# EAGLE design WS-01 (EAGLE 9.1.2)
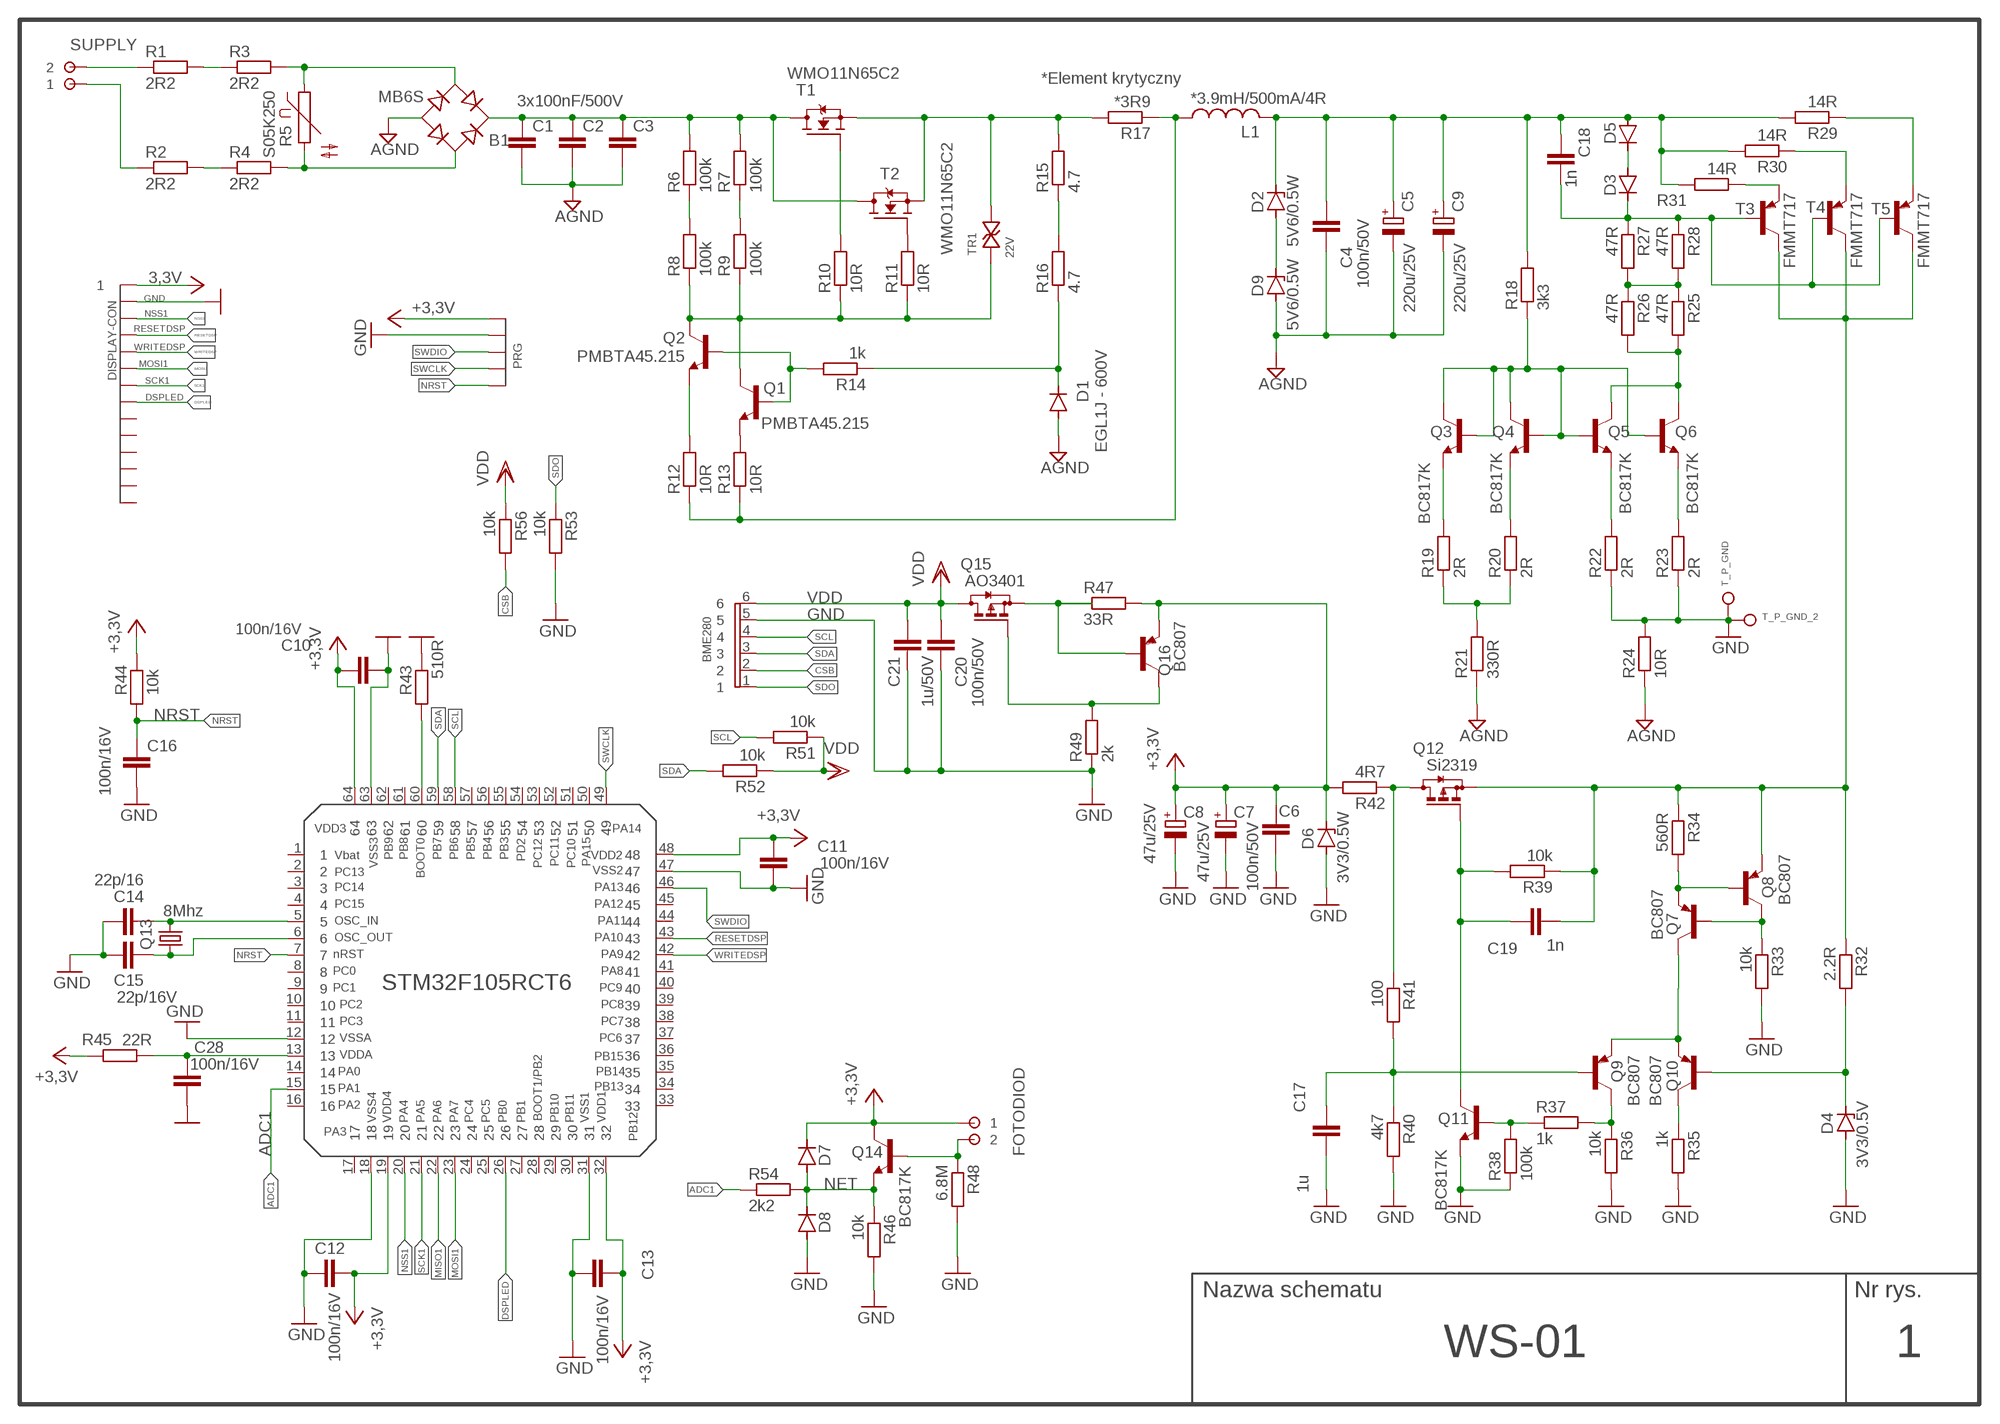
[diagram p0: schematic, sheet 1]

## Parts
B1  MB6S  [SOIC-4]
BME280  GOLDPIN6  [GOLDPIN6]
C1  3x100nF/500V  C-EUC1812  [C1812]
C2  C-EUC1812  [C1812]
C3  C-EUC1812  [C1812]
C4  100n/50V  C-EUC0805  [C0805]
C5  220u/25V  CPOL-EU175TMP-0810  [175TMP-0810]
C6  100n/50V  C-EUC0805  [C0805]
C7  47u/25V  CPOL-EU153CLV-0505  [153CLV-0505]
C8  47u/25V  CPOL-EU153CLV-0505  [153CLV-0505]
C9  220u/25V  CPOL-EU175TMP-0810  [175TMP-0810]
C10  100n/16V  C-EUC0805  [C0805]
C11  100n/16V  C-EUC0805  [C0805]
C12  100n/16V  C-EUC0805  [C0805]
C13  100n/16V  C-EUC0805  [C0805]
C14  22p/16  C-EUC0805  [C0805]
C15  22p/16V  C-EUC0805  [C0805]
C16  100n/16V  C-EUC0805  [C0805]
C17  1u  C-EUC0805  [C0805]
C18  1n  C-EUC0805  [C0805]
C19  1n  C-EUC0805  [C0805]
C20  100n/50V  C-EUC0805  [C0805]
C21  1u/50V  C-EUC0805  [C0805]
C28  100n/16V  C-EUC0805  [C0805]
D1  EGL1J - 600V  DIODE-MINIMELF  [MINIMELF]
D2  5V6/0.5W  ZENER-DIODESOD80C  [SOD80C]
D3  DIODE-MINIMELF  [MINIMELF]
D4  3V3/0.5V  ZENER-DIODESOD80C  [SOD80C]
D5  DIODE-MINIMELF  [MINIMELF]
D6  3V3/0.5W  ZENER-DIODESOD80C  [SOD80C]
D7  DIODE-MINIMELF  [MINIMELF]
D8  DIODE-MINIMELF  [MINIMELF]
D9  5V6/0.5W  ZENER-DIODESOD80C  [SOD80C]
DISPLAY-CON  GOLDPIN14  [GOLDPIN14]
FOTODIOD  ARK254  [ARK254]
L1  *3.9mH/500mA/4R  L-US6000-XXX-RC  [6000-XXXX-RC]
PRG  GOLDPIN5  [GOLDPIN5]
Q1  PMBTA45.215  BC847ASMD  [SOT23]
Q2  PMBTA45.215  BC847ASMD  [SOT23]
Q3  BC817K  BC817-16LT1SMD  [SOT23-BEC]
Q4  BC817K  BC817-16LT1SMD  [SOT23-BEC]
Q5  BC817K  BC817-16LT1SMD  [SOT23-BEC]
Q6  BC817K  BC817-16LT1SMD  [SOT23-BEC]
Q7  BC807  BC807-25SMD  [SOT23-BEC]
Q8  BC807  BC807-25SMD  [SOT23-BEC]
Q9  BC807  BC807-25SMD  [SOT23-BEC]
Q10  BC807  BC807-25SMD  [SOT23-BEC]
Q11  BC817K  BC817-16LT1SMD  [SOT23-BEC]
Q12  Si2319  BSS84  [SOT23]
Q13  8Mhz  CRYSTALHC49S  [HC49/S]
Q14  BC817K  BC817-16LT1SMD  [SOT23-BEC]
Q15  AO3401  BSS84  [SOT23]
Q16  BC807  BC807-25SMD  [SOT23-BEC]
R1  2R2  R-EU_R0805  [R0805]
R2  2R2  R-EU_R0805  [R0805]
R3  2R2  R-EU_R0805  [R0805]
R4  2R2  R-EU_R0805  [R0805]
R5  S05K250  [S05K250]
R6  100k  R-EU_R1206  [R1206]
R7  100k  R-EU_R1206  [R1206]
R8  100k  R-EU_R1206  [R1206]
R9  100k  R-EU_R1206  [R1206]
R10  10R  R-EU_R0805  [R0805]
R11  10R  R-EU_R0805  [R0805]
R12  10R  R-EU_R0805  [R0805]
R13  10R  R-EU_R0805  [R0805]
R14  1k  R-EU_R1206  [R1206]
R15  4.7  R-EU_R0805  [R0805]
R16  4.7  R-EU_R0805  [R0805]
R17  *3R9  R-EU_R1206  [R1206]
R18  3k3  R-EU_R0805  [R0805]
R19  2R  R-EU_R0805  [R0805]
R20  2R  R-EU_R0805  [R0805]
R21  330R  R-EU_R0805  [R0805]
R22  2R  R-EU_R0805  [R0805]
R23  2R  R-EU_R0805  [R0805]
R24  10R  R-EU_R1206  [R1206]
R25  47R  R-EU_R1206  [R1206]
R26  47R  R-EU_R1206  [R1206]
R27  47R  R-EU_R1206  [R1206]
R28  47R  R-EU_R1206  [R1206]
R29  14R  R-EU_R0805  [R0805]
R30  14R  R-EU_R0805  [R0805]
R31  14R  R-EU_R0805  [R0805]
R32  2.2R  R-EU_R0805  [R0805]
R33  10k  R-EU_R0805  [R0805]
R34  560R  R-EU_R0805  [R0805]
R35  1k  R-EU_R0805  [R0805]
R36  10k  R-EU_R0805  [R0805]
R37  1k  R-EU_R0805  [R0805]
R38  100k  R-EU_R0805  [R0805]
R39  10k  R-EU_R0805  [R0805]
R40  4k7  R-EU_R0805  [R0805]
R41  100  R-EU_R0805  [R0805]
R42  4R7  R-EU_R1206  [R1206]
R43  510R  R-EU_R0805  [R0805]
R44  10k  R-EU_R0805  [R0805]
R45  22R  R-EU_R0805  [R0805]
R46  10k  R-EU_R0805  [R0805]
R47  33R  R-EU_R0805  [R0805]
R48  6.8M  R-EU_R0805  [R0805]
R49  2k  R-EU_R0805  [R0805]
R51  10k  R-EU_R0805  [R0805]
R52  10k  R-EU_R0805  [R0805]
R53  10k  R-EU_R0805  [R0805]
R54  2k2  R-EU_R0805  [R0805]
R56  10k  R-EU_R0805  [R0805]
SUPPLY  ARK254  [ARK254]
T1  WMO11N65C2  MOS_TO252  [MOS_TO252]
T2  WMO11N65C2  MOS_TO252  [MOS_TO252]
T3  FMMT717  BC807-16-PNP-SOT23-BEC  [SOT23-BEC]
T4  FMMT717  BC807-16-PNP-SOT23-BEC  [SOT23-BEC]
T5  FMMT717  BC807-16-PNP-SOT23-BEC  [SOT23-BEC]
T_P_GND  PAD3  [PAD3]
T_P_GND_2  PAD3  [PAD3]
TR1  22V  SMAJ30CA-TR__DO214AC+MINIMELF  [DO214AC+MINIMELF_BIDIR]
U$2  STM32F105RCT6  [STM32F105RCT6]

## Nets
ADC1: R54.1 U$2.15
AGND: B1.- C1.2 C2.2 C3.2 C4.2 C5.- C9.- D1.A D9.A R21.1 R24.1
CSB: BME280.2 R56.2
DSPLED: DISPLAY-CON.8 U$2.26
GND: BME280.5 C6.2 C7.- C8.- C10.1 C11.1 C12.1 C13.2 C14.1 C15.1 C16.2 C17.2 C20.2 C21.2 C28.1 D4.A D6.A D8.A DISPLAY-CON.2 PRG.2 Q11.E R22.1 R23.1 R24.2 R33.2 R35.2 R36.2 R38.1 R40.2 R43.2 R46.2 R48.2 R49.1 R53.2 T_P_GND.P T_P_GND_2.P U$2.12 U$2.18 U$2.31 U$2.47 U$2.63
MISO1: U$2.22
MOSI1: DISPLAY-CON.6 U$2.23
N$1: R1.1 SUPPLY.2
N$2: R2.1 SUPPLY.1
N$3: R1.2 R3.1
N$4: R2.2 R4.1
N$5: B1.~2(AC2) R3.2 R5.1
N$6: B1.~1(AC1) R4.2 R5.2
N$7: B1.+ C1.1 C2.1 C3.1 R6.2 R7.2 T1.2(D) T2.2(D)
N$8: R6.1 R8.2
N$9: R7.1 R9.2
N$10: R15.2 R17.2 T1.3(S) T2.3(S) TR1.P$2
N$11: R11.2 T2.1(G)
N$12: Q1.3(C) Q2.3(C) R8.1 R9.1 R10.1 R11.1 TR1.P$1
N$13: Q1.1(B) Q2.1(B) R14.2
N$14: R10.2 T1.1(G)
N$15: Q1.2(E) R13.2
N$16: Q2.2(E) R12.2
N$17: L1.1 R12.1 R13.1 R17.1
N$18: R30.1 T4.E
N$19: R15.1 R16.2
N$20: D1.C R14.1 R16.1
N$21: D3.A D5.C
N$22: C4.1 C5.+ C9.+ C18.1 D2.C D5.A L1.2 R18.2 R29.2 R30.2 R31.2
N$23: Q5.C Q6.C R25.2 R26.2
N$24: Q3.E R19.2
N$25: Q4.E R20.2
N$26: R19.1 R20.1 R21.2
N$27: Q3.B Q3.C Q4.B Q4.C Q5.B Q6.B R18.1
N$28: Q15.2(S) Q16.B R47.1
N$29: R25.1 R26.1 R27.2 R28.2
N$30: Q5.E R22.2
N$31: Q6.E R23.2
N$32: C18.2 D3.C R27.1 R28.1 T3.B T4.B T5.B
N$33: R29.1 T5.E
N$34: R31.1 T3.E
N$35: D4.C Q10.B R32.2
N$36: Q7.B Q8.C R33.1
N$37: Q10.C R35.1
N$38: Q9.C R36.1 R37.2
N$39: Q7.E Q8.B R34.2
N$40: C19.2 Q8.E Q12.2(S) R32.1 R34.1 R39.1 T3.C T4.C T5.C
N$41: Q11.B R37.1 R38.2
N$42: C19.1 Q11.C Q12.1(G) R39.2
N$43: Q7.C Q9.E Q10.E
N$44: C14.2 Q13.2 U$2.5
N$45: Q12.3(D) R41.1 R42.1
N$46: C17.1 Q9.B R40.1 R41.2
N$47: C15.2 Q13.1 U$2.6
N$48: R43.1 U$2.60
N$49: C28.2 R45.1 U$2.13
N$50: Q15.1(G) Q16.C R49.2
N$51: FOTODIOD.2 Q14.B R48.1
N$52: D2.A D9.C
NET: D7.A D8.C Q14.E R46.1 R54.2
NRST: C16.1 PRG.5 R44.1 U$2.7
NSS1: DISPLAY-CON.3 U$2.20
RESETDSP: DISPLAY-CON.4 U$2.43
SCK1: DISPLAY-CON.7 U$2.21
SCL: BME280.4 R51.2 U$2.58
SDA: BME280.3 R52.2 U$2.59
SDO: BME280.1 R53.1
SWCLK: PRG.4 U$2.49
SWDIO: PRG.3 U$2.46
VCC: C6.1 C7.+ C8.+ C10.2 C11.2 C12.2 C13.1 D6.C D7.C DISPLAY-CON.1 FOTODIOD.1 PRG.1 Q14.C Q16.E R42.2 R44.2 R45.2 R47.2 U$2.19 U$2.32 U$2.48 U$2.64 ; supply symbol labelled +3,3V, 3,3V
VDD: BME280.6 C20.1 C21.1 Q15.3(D) R51.1 R52.1 R56.1
WRITEDSP: DISPLAY-CON.5 U$2.42
Unconnected: DISPLAY-CON.9 DISPLAY-CON.10 DISPLAY-CON.11 DISPLAY-CON.12 DISPLAY-CON.13 DISPLAY-CON.14 U$2.1 U$2.2 U$2.3 U$2.4 U$2.8 U$2.9 U$2.10 U$2.11 U$2.14 U$2.16 U$2.17 U$2.24 U$2.25 U$2.27 U$2.28 U$2.29 U$2.30 U$2.33 U$2.34 U$2.35 U$2.36 U$2.37 U$2.38 U$2.39 U$2.40 U$2.41 U$2.44 U$2.45 U$2.50 U$2.51 U$2.52 U$2.53 U$2.54 U$2.55 U$2.56 U$2.57 U$2.61 U$2.62

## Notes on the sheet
- *Element krytyczny
- WS-01 | 1

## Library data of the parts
B1 = rectifier:MB*S: Bridge Rectifier Source: http://www.fairchildsemi.com/ds/MB/MB6S.pdf
BME280 = GOLDPIN6:GOLDPIN6
C1-C3 = resistor:C-EU: CAPACITOR, European symbol
C4 C6 C10-C21 C28 = rcl:C-EU: CAPACITOR, European symbol; SPICEPREFIX: C
C5 C9 = rcl:CPOL-EU: POLARIZED CAPACITOR, European symbol; SPICEPREFIX: C
C7 C8 = resistor:CPOL-EU: POLARIZED CAPACITOR, European symbol
D1 D3 D5 D7 D8 = diode:DIODE-: DIODE
D2 D4 D6 D9 = diode:ZENER-DIODE: Z-Diode
DISPLAY-CON = Goldpin14:GOLDPIN14: 3 Goldpin
FOTODIOD SUPPLY = ark254:ARK254
L1 = rcl:L-US: INDUCTOR, American symbol; SPICEPREFIX: L
PRG = Goldpin5:GOLDPIN5: 3 Goldpin
Q1 Q2 = transistor-npn:BC847*: NPN Transistor
Q3-Q6 Q11 Q14 = transistor-npn:BC817*: NPN Transistor
Q7-Q10 Q16 = transistor-pnp:BC807*: PNP Transistror
Q12 Q15 = transistor-small-signal:BSS84: P-CHANNEL MOS FET
Q13 = crystal:CRYSTAL: CRYSTAL; OC_FARNELL: 1667008; OC_NEWARK: unknown
R1-R4 R6-R23 R25-R49 R51-R54 R56 = rcl:R-EU_: RESISTOR, European symbol; SPICEPREFIX: R
R5 = varistor:S05K250: VARISTOR
R24 = resistor:R-EU_: RESISTOR, European symbol
T1 T2 = MOS_TO252:MOS_TO252
T3-T5 = transistor:*-PNP-: PNP Transistror
T_P_GND T_P_GND_2 = PAD3:PAD3
TR1 = transil:SMAJ30CA-TR__DO214AC+MINIMELF: Transil SMAJ 30 Volt BIDIR.
U$2 = STM32F105RBT6:STM32F105RCT6

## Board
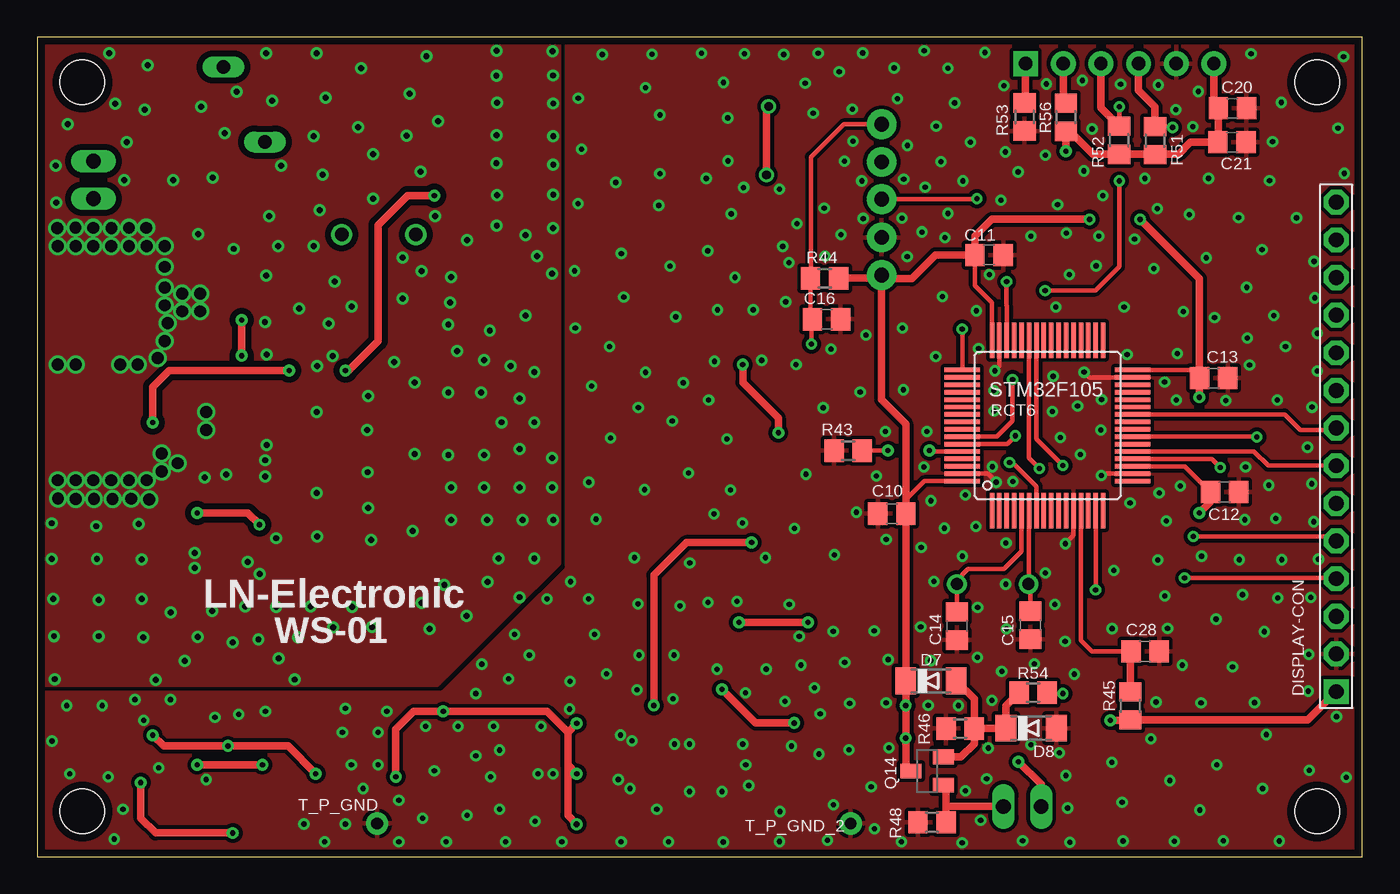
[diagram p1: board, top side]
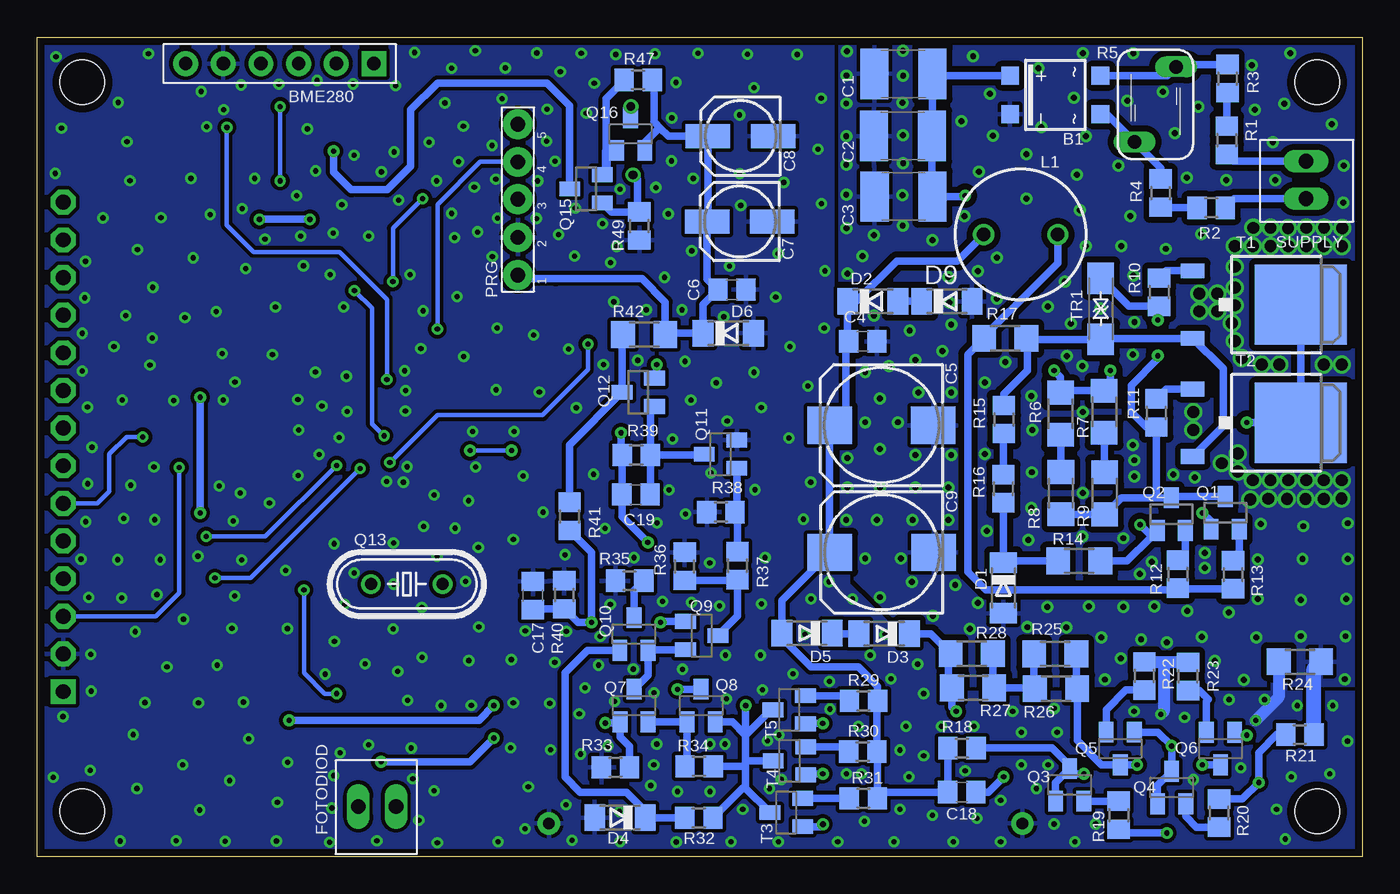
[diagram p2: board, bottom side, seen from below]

Size 89.4 x 55.3 mm. Coordinates in mm from the lower left corner, seen from the top.
Outline: 0,0 89.4,0 89.4,55.3 0,55.3 0,0
Copper layers (1*16): Top 0.035mm / dielectric 1.5mm / Bottom 0.035mm
Design rules "default *": minimum track width 6mil, minimum drill 0.35mm, track to track 6mil, track to pad 6mil, pad to pad 6mil, via to via 6mil, smd to smd 6mil, copper to edge 20mil, drill to drill 6mil, minimum pad ring 10mil, minimum via ring 8mil, stop-mask expansion 4mil, vias tented up to drill 50mil, thermal gap 10mil
Holes 3 mm at 3.05,52.25 3.05,3.05 86.35,3.05 86.35,52.25

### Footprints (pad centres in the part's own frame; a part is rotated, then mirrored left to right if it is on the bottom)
SOIC-4 = smd 1.2 x 1.2: + 1.3,3.05; - -1.3,3.05; ~1 -1.3,-3.05; ~2 1.3,-3.05
GOLDPIN6 = drill 0.9 pad 1.676 square: 1 0,0 | drill 0.9 pad 1.676: 2 2.54,0; 3 5.08,0; 4 7.62,0; 5 10.16,0; 6 12.7,0
C1812 = smd 1.9 x 3.4: 1 -1.95,0; 2 1.95,0
C0805 = smd 1.3 x 1.5: 1 -0.95,0; 2 0.95,0
175TMP-0810 = smd 3 x 2.5: + 3.5,0; - -3.5,0
153CLV-0505 = smd 3 x 1.6: + 2.2,0; - -2.2,0
MINIMELF = smd 1.4 x 1.8: A 1.7,0; C -1.7,0
SOD80C = smd 1.4 x 1.8: A 1.7,0; C -1.7,0
GOLDPIN14 = drill 1 pad 1.676 square: 1 0,0 | drill 1 pad 1.676 octagon: 2 2.54,0; 3 5.08,0; 4 7.62,0; 5 10.16,0; 6 12.7,0; 7 15.24,0; 8 17.78,0; 9 20.32,0; 10 22.86,0; 11 25.4,0; 12 27.94,0; 13 30.48,0; 14 33.02,0
ARK254 = drill 1 long: 1 -0.06,0; 2 2.48,0
6000-XXXX-RC = drill 0.9 pad 1.422: 1 -2.5,0; 2 2.5,0
GOLDPIN5 = drill 1 pad 2: 1 0,0.01; 2 2.54,0.01; 3 5.12,0.01; 4 7.64,0.01; 5 10.18,0.01
SOT23 = smd 1 x 1.4: 1 -0.95,-1.1; 2 0.95,-1.1; 3 0,1.1
SOT23-BEC = smd 1 x 1.4: B -0.95,-1.1; C 0,1.1; E 0.95,-1.1
HC49/S = drill 0.813: 1 -2.413,0; 2 2.413,0
R0805 = smd 1.3 x 1.5: 1 -0.95,0; 2 0.95,0
S05K250 = drill 0.914 long: 1 -1.397,-2.54; 2 1.397,2.54
R1206 = smd 1.6 x 1.803: 1 -1.422,0; 2 1.422,0
MOS_TO252 = smd 1 x 1.6: 1 -2.28,-2.26; 3 2.28,-2.26 | smd 5.4 x 6.2: 2 0,5.04
PAD3 = drill 0.8 pad 1.5: P 0,0
DO214AC+MINIMELF_BIDIR = smd 2.123 x 1.8: P$1 -2.064,0; P$2 2.064,0
STM32F105RCT6 = smd 0.3 x 2.4: 1 0,0; 2 0.5,0; 3 1,0; 4 1.5,0; 5 2,0; 6 2.5,0; 7 3,0; 8 3.5,0; 9 4,0; 10 4.5,0; 11 5,0; 12 5.5,0; 13 6,0; 14 6.5,0; 15 7,0; 16 7.5,0; 33 7.5,11.5; 34 7,11.5; 35 6.5,11.5; 36 6,11.5; 37 5.5,11.5; 38 5,11.5; 39 4.5,11.5; 40 4,11.5; 41 3.5,11.5; 42 3,11.5; 43 2.5,11.5; 44 2,11.5; 45 1.5,11.5; 46 1,11.5; 47 0.5,11.5; 48 0,11.5 | smd 2.4 x 0.3: 17 9.5,2; 18 9.5,2.5; 19 9.5,3; 20 9.5,3.5; 21 9.5,4; 22 9.5,4.5; 23 9.5,5; 24 9.5,5.5; 25 9.5,6; 26 9.5,6.5; 27 9.5,7; 28 9.5,7.5; 29 9.5,8; 30 9.5,8.5; 31 9.5,9; 32 9.5,9.5; 49 -2,9.5; 50 -2,9; 51 -2,8.5; 52 -2,8; 53 -2,7.5; 54 -2,7; 55 -2,6.5; 56 -2,6; 57 -2,5.5; 58 -2,5; 59 -2,4.5; 60 -2,4; 61 -2,3.5; 62 -2,3; 63 -2,2.5; 64 -2,2

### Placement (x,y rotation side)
B1  20.72,51.39 90 bottom
BME280  66.68,53.51 180 bottom
C1  30.96,52.82 180 bottom
C2  30.99,48.63 180 bottom
C3  30.95,44.53 180 bottom
C4  33.7,34.77 0 bottom
C5  32.45,29.11 180 bottom
C6  42.53,38.26 0 bottom
C7  42,42.85 180 bottom
C8  41.95,48.62 180 bottom
C9  32.42,20.53 180 bottom
C10  57.66,23.15 0 top
C11  64.22,40.6 180 top
C12  80.1,24.61 180 top
C13  79.36,32.29 0 top
C14  62.05,15.56 90 top
C15  67,15.62 90 top
C16  53.26,36.26 0 top
C17  55.96,17.62 90 bottom
C18  27.02,4.36 0 bottom
C19  49.01,24.44 180 bottom
C20  80.63,50.49 0 top
C21  80.6,48.2 0 top
C28  74.74,13.86 180 top
D1  24.22,18.13 270 bottom
D2  33.03,37.47 0 bottom
D3  32.26,15.04 180 bottom
D4  50.08,2.64 180 bottom
D5  37.46,15.08 180 bottom
D6  42.77,35.32 0 bottom
D7  60.29,11.87 0 top
D8  67.05,8.67 0 top
D9  28.03,37.47 0 bottom
DISPLAY-CON  87.63,11.14 90 top
FOTODIOD  67.67,3.39 0 bottom
L1  23.05,41.98 180 bottom
PRG  56.96,39.24 90 bottom
Q1  9.26,23.2 0 bottom
Q2  12.89,23.12 0 bottom
Q3  19.75,4.85 0 bottom
Q4  12.87,4.67 0 bottom
Q5  16.34,7.3 180 bottom
Q6  9.57,7.3 180 bottom
Q7  49.14,10.2 0 bottom
Q8  44.6,10.21 0 bottom
Q9  44.57,14.92 270 bottom
Q10  49.14,15.03 0 bottom
Q11  43.3,27.16 90 bottom
Q12  48.84,31.33 90 bottom
Q13  64.46,18.39 0 bottom
Q14  60.04,5.78 90 top
Q15  52.37,45.06 90 bottom
Q16  49.36,48.76 0 bottom
R1  9.15,48.34 90 bottom
R2  10.2,43.78 180 bottom
R3  9.1,52.5 90 bottom
R4  13.61,44.77 90 bottom
R5  13.96,50.75 180 bottom
R6  20.36,29.89 90 bottom
R7  17.42,30.02 90 bottom
R8  20.34,24.54 90 bottom
R9  17.39,24.52 90 bottom
R10  13.71,38.09 90 bottom
R11  13.91,29.94 90 bottom
R12  12.45,19.07 90 bottom
R13  8.72,19.03 90 bottom
R14  19.11,19.96 0 bottom
R15  24.18,29.5 90 bottom
R16  24.22,24.83 90 bottom
R17  24.1,34.98 0 bottom
R18  27.01,7.33 180 bottom
R19  16.44,2.8 90 bottom
R20  9.67,2.95 270 bottom
R21  4.22,8.24 180 bottom
R22  14.7,12.19 270 bottom
R23  11.77,12.16 270 bottom
R24  4.22,13.16 180 bottom
R25  20.73,13.68 0 bottom
R26  20.67,11.34 0 bottom
R27  26.26,11.4 0 bottom
R28  26.35,13.7 0 bottom
R29  33.65,10.52 0 bottom
R30  33.7,7.09 0 bottom
R31  33.67,3.94 0 bottom
R32  44.76,2.62 180 bottom
R33  50.38,6.03 180 bottom
R34  44.74,6.09 180 bottom
R35  49.43,18.62 180 bottom
R36  45.72,19.59 90 bottom
R37  42.15,19.64 270 bottom
R38  43.27,23.25 0 bottom
R39  48.98,27.1 0 bottom
R40  53.84,17.67 90 bottom
R41  53.48,22.96 270 bottom
R42  48.45,35.22 0 bottom
R43  54.71,27.39 180 top
R44  53.12,39.02 0 top
R45  73.74,10.18 270 top
R46  62.27,8.65 180 top
R47  48.86,52.41 0 bottom
R48  60.36,2.33 180 top
R49  48.78,42.55 90 bottom
R51  75.41,48.31 90 top
R52  72.99,48.34 90 top
R53  66.61,49.91 270 top
R54  67.19,11.07 180 top
R56  69.39,49.89 90 top
SUPPLY  3.81,44.45 90 bottom
T1  9.19,37.25 270 bottom
T2  9.19,29.28 270 bottom
T3  38.85,2.98 90 bottom
T4  38.65,6.47 90 bottom
T5  38.67,9.92 90 bottom
T_P_GND  22.93,2.24 0 top
T_P_GND_2  54.88,2.24 0 top
TR1  17.65,36.96 270 bottom
U$2  64.41,23.34 0 top

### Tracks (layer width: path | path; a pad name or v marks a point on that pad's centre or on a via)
ADC1  (via drill 0.35 pad 0.35)
  Top 0.3: U$2.15 v71.41,18.01 v71.4,18 | v69.2,11 68.21,11 R54.1
  Bottom 0.3: v71.4,18 71.4,12.4 70,11 v69.2,11
AGND  (via drill 0.4, 0.8)
  Bottom 0.813: 3.27,12.68 R24.1
  Bottom 1.016: R21.1 3.27,12.68
  other vias: 1.4,25.4 2.6,25.4 3.8,25.4 5,25.4 6.2,25.4 7.4,25.4 8.4,26 8.4,27.2 6.8,33.2 5.6,33.2 2.6,33.2 1.4,33.2 1.4,41.2 2.6,41.2 3.8,41.2 5,41.2 6.2,41.2 7.4,41.2 8.6,41.2 11,38 11,36.8 11.4,30 11.4,28.8 9.8,38 9.8,36.8 8.8,36 8.6,37.2 8.6,38.4 8.6,39.8 8.6,34.8 8.13,33.64 9.49,26.55 10.62,20.49 10.62,19.49 14.22,19.89 15.02,19.09 16.13,21.49 18.88,21.61 22.34,23.52 22.54,21.37 25.34,21.97 18.87,24.55 22.31,25.94 22.27,28.78 22.33,31.07 18.87,29.99 11.31,25.59 12.77,25.78 15.49,27.78 15.4,25.66 25.47,27.18 25.47,31.98 24.07,33.38 21.21,37.13 27.87,37.38 19.67,35.98 17.67,36.98 15.37,36.06 20.06,38.81 18.66,41.21 15.46,39.21 13.26,41.01 10.86,42.01 15.66,43.21 16.46,46.61 18.66,48.61 19.26,46.01 19.06,43.61 22.66,44.41 25.86,46.21 27.06,49.61 22.66,47.41 26.86,43.21 24.66,40.41 21.66,49.21 19.46,51.21 21.86,53.21 26.26,54.01 18.86,54.21 15.46,54.21 15.86,51.01 12.66,48.81 11.86,45.81 9.19,45.64 11.06,50.61 13.46,51.61 6.06,48.21 7.26,50.41 7.46,53.41 4.86,54.21 5.26,50.81 2.06,49.41 1.26,46.61 5.89,45.65 1.28,44.12 16.26,41.21 15.5,33.89 18.9,33.09 19.95,33.78 25.94,39.51 27.74,35.91 27.94,39.11 32.94,36.51 28.34,34.11 27.74,31.31 29.94,31.31 30.54,35.51 31.94,33.11 33.54,32.71 32.54,30.91 30.14,33.51 31.34,29.31 33.54,29.31 32.54,27.51 27.74,27.11 30.14,27.11 34.74,26.91 34.74,24.91 32.54,24.91 30.14,24.91 27.94,24.91 27.94,22.71 30.34,22.71 32.74,22.71 34.82,22.71 33.54,20.11 31.14,20.11 32.54,17.51 30.4,18.53 25.94,17.11 28.96,16.24 26.48,15.37 27.47,18.34 22.59,15.49 21.24,16.86 19.98,15.48 18.46,16.9 17.62,14.8 17.37,11.95 16.3,13.37 14.93,14.65 13.19,14.45 16.12,16.85 14.05,16.88 11.8,16.58 10.84,14.82 9.95,13.21 8.01,11.93 7.17,14.8 9.01,16.48 4.16,14.88 7.07,17.38 4.16,17.32 1.18,11.98 1.14,14.88 1.08,17.4 0.99,20.1 4.04,20.08 7.07,20.06 0.99,22.5 3.99,22.3 6.86,22.44 15.38,26.75 29.02,41.61 33.72,40.52 24.66,37.67 34.74,39.33 32.95,41.93 34.82,44.66 31.01,42.58 31.03,44.64 30.98,46.8 31,48.69 31.03,50.87 30.98,52.68 31,54.39 34.77,54.34 34.8,52.71 34.82,50.82 34.82,48.6 34.82,46.7 34.8,42.42 24.92,48.66 25.13,51.49 1.41,24.16 2.61,24.14 3.84,24.14 5.09,24.14 6.34,24.15 7.56,24.1 1.37,42.41 2.59,42.44 3.79,42.43 5.02,42.4 6.2,42.43 7.35,42.43
  pour Top (isolate 0.406): 0.4,11.6 27,11.6 31.8,16.4 35.2,19.8 35.2,55 0.4,55
  pour Bottom (isolate 0.406): 0.4,11.6 27,11.6 31.8,16.4 35.2,19.8 35.2,55 0.4,55
CSB
  Top 0.508: BME280.2 69.22,51.01 R56.2
DSPLED
  Top 0.3: U$2.26 84.16,29.84 85.2,28.8 87.51,28.8 DISPLAY-CON.8
GND  (via drill 0.35)
  Top 0.3: U$2.18 71.9,25.84 v71.78,25.72 | U$2.63 64.12,25.84 v64.69,25.27 | U$2.31 70.97,32.34 v70.62,32.69 | U$2.47 64.91,33.09 v64.6,32.78 | U$2.12 69.91,21.66 v69.37,21.12
  Bottom 0.3: 14.67,13.11 R22.1 | 13.4,9.8 v13.6,9.6
  Bottom 0.813: R23.1 13.4,13.11 | 13.4,13.11 14.67,13.11 | 13.4,13.11 13.4,9.8 | R24.2 5.64,10.76 v7.2,9.2
  other vias: 5.2,1.2 5.8,3.2 4.8,5.4 2.2,5.6 1,7.8 2,10.2 8.2,6 11.4,5.2 4.4,10.2 9,10.6 12,9.4 15.4,9.8 6.6,10.6 20.8,10 20.6,8.4 23,8.4 23.6,9.8 26.2,8.8 28.4,8.8 30.8,8.8 31.2,7.2 29.6,6.8 30.6,5.4 26.8,5.8 21.2,6.2 23,6.2 22,4.6 24.4,3.8 20.8,2.2 18,2.2 19.4,1 24.4,1 26,2.6 27.6,1 29,2.8 31.2,3.2 31.6,1 33.6,2.4 35.4,1 42.6,1 40,4.6 39.2,5.2 33.8,5.6 34.8,5.6 34,8.8 35.92,9.96 39.36,8.21 40.13,7.81 41.8,3.2 39.4,1 44,4.4 46.2,4.4 48,4.8 47.6,7.6 47.8,6.2 44,7.6 43,7.6 29.6,11 31.8,12 30,13 33.2,13.6 32.2,15 34.4,17.4 37.2,17.4 37.6,15 35.96,11.84 38.41,12.33 40.6,13.6 40.47,11.26 42.96,13.6 42.9,10.66 45.86,12.65 47.79,11.06 49.18,12.66 51.52,12.93 50.45,10.48 52.83,9.63 50.89,7.46 52.74,6.93 50.11,3.05 50.07,1.03 46.29,0.99 53.71,3.5 53.31,1.1 51.41,14.87 53.7,15.21 54.48,13.12 56.46,15.24 57.41,13.3 57.27,10.38 54.81,10.34 54.76,7.22 57.47,7.35 56.27,4.72 56.48,1.88 58.31,1.01 62.4,0.95 63.65,2.45 66.48,1.07 64.05,5.25 62.62,4.44 69.67,0.98 69.39,5.47 68.95,7 64.16,7.33 67.04,7.54 73.26,1.06 69.51,3.29 73.19,3.68 72.5,6.37 75.12,7.95 76.41,5.14 76.72,1.05 80.01,1.08 83.8,1.06 78.43,3.15 82.66,4.6 79.58,6.2 82.91,8.24 85.81,5.82 87.65,9.46 88.31,5.36 75.48,10.43 78.51,10.38 82.12,10.4 85.74,11.17 85.79,13.66 82.78,15.19 79.53,16.03 77.26,12.92 76.07,17.6 72.51,15.39 72.63,19.32 75.59,20.02 78.55,20.27 81.09,20.04 83.96,20.04 86.44,20.07 85.92,17.5 83.69,17.47 81.31,17.68 73.73,23.86 76.18,22.66 77.12,25.02 70.37,27.13 69.03,28.29 68.48,30.03 68.54,32.41 71.81,30.85 71.75,28.78 70.19,30.4 64.56,30.07 64.55,31.46 64.44,26.31 65.82,25.31 75.69,24.55 60.29,24.02 62.61,24.41 59.63,20.87 61.21,22.17 63.32,22.29 65.36,21.17 62.41,20.28 60.5,18.57 59.6,15.51 60.28,13.23 60.11,10.22 62.14,10.2 64.4,10.54 65.07,12.5 63.43,13.44 65.39,15.37 63.45,16.82 65.34,18.39 68.01,19.15 68.66,17.02 69.34,14.52 67.27,13.02 69.96,12.32 81.46,22.74 86.12,22.6 83.56,22.82 83.09,25.06 81.52,26.3 85.99,25.16 85.7,27.62 86,30.33 80.19,30.77 83.65,30.82 81.79,33.17 86.35,32.76 84.21,34.41 86.35,35.31 81.64,35 79.42,36.38 83.42,36.5 86.19,37.7 81.59,38.41 86.14,40.17 82.63,40.96 78.86,40.4 77.72,43.33 81.05,43.12 84.95,43.1 88.18,46.1 83.14,45.62 79.02,45.77 83.34,48.24 87.75,49.16 83.93,50.89 81.89,54.18 88.13,53.97 77.96,49.25 78.33,51.63 75.63,52.07 76.82,50.4 73.09,52.11 70.5,52.37 68.08,52.14 65.21,52.02 63.94,54.26 61.44,53.2 71.16,49.1 68.01,47.33 66.18,46.2 65.31,47.55 70.61,46.27 71.89,44.6 74.73,45.77 75.57,43.73 68.84,44 65.01,44.29 62.46,45.6 62.96,48.2 61.9,50.86 58.04,51.14 58.7,47.99 54.99,50.43 57.81,53.22 54.1,52.97 52.35,50.17 51.82,52.18 50.36,54.12 55.69,54.22 59.84,54.37 52.69,54.2 60.97,46.9 60.65,49.28 55.03,48.27 55.63,45.59 54.46,46.93 58.46,45.71 59.91,45.18 50.08,45.04 61.44,43.41 61.23,41.77 58.69,40.49 58.34,43.09 59.68,42.15 55.72,43.06 53.1,43.75 53.15,40.53 54.23,41.98 51.26,42.71 50.3,41.18 50.71,40.09 47.08,39.09 45.9,36.9 45.24,40.88 46.82,43.37 45.14,45.77 46.6,46.95 47.66,45.15 46.59,49.84 46.31,52.24 47.71,54.17 44.81,54.2 41.48,54.15 38.12,54.12 36.51,51.17 41.04,51.88 42.01,50.05 36.72,47.73 36.49,44.06 42.01,46.08 41.93,43.94 39.03,45.49 36.26,39.53 39.41,40.7 42.7,39.84 36.31,35.66 39.57,37.75 43.08,36.42 45.7,33.42 48.88,33.49 50.5,37.44 48.31,36.9 51.2,33.2 53.55,34.25 55.91,35.2 55.52,31.35 58.43,31.5 60.62,33.75 58.38,35.67 61.06,37.79 63.37,36.83 63.51,34.28 37.41,31.76 41.05,32.68 45.3,30.81 46.53,28.18 42.84,29.39 38.69,28.24 37.22,25.27 40.98,24.76 38.62,34.41 40.55,30.3 43.59,31.97 43.95,25.89 46.77,24.74 45.66,23.13 47.59,22.51 44.02,19.82 49.13,20.18 51.09,22.15 51.87,25.8 37.7,22.77 40.29,20.18 40.54,17.06 35.98,18.56 43.37,16.93 47.21,17.22 50.73,17.03 53.79,20.37 57.27,21.4 55.27,23.24 56.61,25.68 45.25,17.16 80.64,12.81 76.26,15.41 52.43,11.4 73.52,33.88 76.91,33.94 77.31,36.78 75.32,39.68 68.72,37.08 73.32,37.08 76.05,32.02 76.85,30.82 60.03,28.69 59.83,26.29 57.23,28.69 53.03,30.29 64.23,39.27 67.03,41.87 71.63,41.87 69.43,42.07 74.03,41.67 69.63,39.27 71.43,39.87
  pour Bottom (isolate 0.254, rank 2): 0,11.6 26.4,11.6 34.8,20 34.8,55.2 89.25,55.2 89.25,0.12 0,0.12
  pour Top (isolate 0.254, rank 2): 0,11.6 26.4,11.6 34.8,20 34.8,55.2 89.25,55.2 89.25,0.12 0,0.12
MOSI1  (via drill 0.35 pad 0.35)
  Top 0.3: U$2.23 82.25,28.34 v82.27,28.32
  Bottom 0.3: v82.27,28.32 83.37,28.32 84.52,27.17 84.52,24.65 85.33,23.84 DISPLAY-CON.6
N$1
  Bottom 0.508: SUPPLY.2 8.69,46.93 R1.1
N$2
  Bottom 0.508: SUPPLY.1 8.64,44.39 R2.1
N$3
  Bottom 0.508: R1.2 9.15,51.49 R3.1
N$4
  Bottom 0.508: R2.2 13.57,43.78 R4.1
N$5
  Bottom 0.508: R3.2 12.41,53.45 R5.1 13.16,52.69 B1.~2
N$6
  Bottom 0.508: R4.2 13.61,46.46 R5.2 17.24,50.09 B1.~1
N$7  (via drill 0.35 pad 0.8)
  Top 0.508: v17,32.8 8.9,32.8 7.8,31.7 v7.8,29.3 | v26.8,44.6 25,44.6 23,42.6 23,34.8 21,32.8 v20.8,32.8
  Bottom 0.508: B1.+ 28.88,52.69 C1.1 29.01,48.01 29,48 29.04,48.04 C2.1 29.04,44.58 C3.1 26.86,44.53 v26.8,44.6 | v7.8,29.3 7.78,29.28 T2.2 T1.2 | v17,32.8 17,31.86 R7.2 20.24,31.44 R6.2 20.36,32.36 v20.8,32.8
N$8
  Bottom 0.508: R6.1 20.34,28.45 R8.2
N$9
  Bottom 0.508: R7.1 17.42,25.97 R9.2
N$10
  Bottom 0.508: 22.59,34.9 TR1.P$2 17.58,34.97 T1.3 9.4,32.92 9.4,29.05 T2.3 | 22.59,34.9 R17.2 | R15.2 24.18,31.22 22.6,32.8 22.6,34.89 22.59,34.9
N$11
  Bottom 0.508: T2.1 13.24,31.56 R11.2
N$12  (via drill 0.35 pad 0.8)
  Top 0.508: v13.8,36.2 v13.8,33.8
  Bottom 0.508: TR1.P$1 15.77,37.14 R10.1 13.71,36.29 v13.8,36.2 | Q1.3 12.81,24.3 Q2.3 14,24.22 | 14,24.22 16.27,24.22 R9.1 20.32,23.09 R8.1 | 14,24.22 13.91,24.31 R11.1 14.59,28.99 15.6,30 15.6,31.8 13.8,33.6 v13.8,33.8
N$13  (via drill 0.35 pad 0.8)
  Top 0.508: v10.8,23.2 14.2,23.2 v15,22.4
  Bottom 0.508: 14.32,21.52 15.88,19.96 R14.2 | 14.32,21.52 13.84,22 Q2.1 | Q1.1 10.21,22.61 v10.8,23.2 | v15,22.4 14.32,21.72 14.32,21.52
N$14
  Bottom 0.508: T1.1 13.22,39.53 R10.2
N$15
  Bottom 0.508: Q1.2 8.31,20.39 R13.2
N$16
  Bottom 0.508: Q2.2 11.94,20.53 R12.2
N$17
  Bottom 0.508: R13.1 12.42,18.08 | 12.42,18.08 R12.1 | L1.1 20.55,40.05 22,38.6 25.52,35.08 R17.1 26.6,33.9 26.6,19.2 25.4,18 12.49,18 12.42,18.08
N$18
  Bottom 0.508: R30.1 34.99,7.42 T4.E
N$19
  Bottom 0.508: R16.2 24.21,28.51 R15.1
N$20
  Bottom 0.508: R14.1 24.09,19.96 D1.C R16.1
N$21
  Bottom 0.508: D5.C 35.72,15.04 D3.A
N$22
  Bottom 0.508: L1.2 27.33,40.2 31.4,40.2 34.13,37.47 D2.C 34.73,34.84 C4.1 34.85,34.57 34.85,29.11 C5.+ 35.95,20.56 C9.+ 39.16,17.29 D5.A 39.16,14.76 37.2,12.8 34,12.8 32.7,11.5 R29.2 32.75,10.47 R30.2 32.72,7.05 R31.2 32.3,4.36 C18.1 R18.2
N$23  (via drill 0.35 pad 0.8)
  Top 0.508: v15.2,6.2 v10.8,6.2
  Bottom 0.508: R25.2 19.3,11.4 R26.2 19.25,7.84 17.6,6.2 15.8,6.2 | Q5.C 15.8,6.2 | 15.8,6.2 v15.2,6.2 | v10.8,6.2 Q6.C
N$24
  Bottom 0.508: R19.2 Q3.E | Q3.E
N$25
  Bottom 0.508: R20.2 11.2,2 11.92,2.72 Q4.E
N$26  (via drill 0.35 pad 0.8)
  Top 0.508: v13.2,1.6 8,1.6 7,2.6 v7,5
  Bottom 0.508: R20.1 8.1,3.9 v7,5 7,7.01 5.77,8.24 R21.2 | R19.1 16.19,1.6 v13.2,1.6
N$27  (via drill 0.35 pad 0.8)
  Top 0.508: v12.87,7.47 8.53,7.47 v7.8,8.2 | v18.8,5.6 16.93,7.47 v12.87,7.47 | v12.87,7.47
  Bottom 0.508: Q5.B 13.8,8.4 v12.87,7.47 Q4.C 13.82,4.82 Q4.B | Q6.B 8.42,8.2 v7.8,8.2 | Q3.C 19.65,6.05 | 19.65,6.05 19.5,6.2 19.65,6.05 | 20.1,5.6 v18.8,5.6 | Q3.B 20.7,5 20.1,5.6 | R18.1 20.93,7.33 19.65,6.05 | 20.1,5.6 19.65,6.05
N$28
  Bottom 0.508: Q16.B 51.02,47.66 51.02,51.13 49.81,52.34 R47.1
  Bottom 0.61: Q16.B 50.98,47.66 50.98,46.3 Q15.2
N$29
  Bottom 0.508: R28.2 24.93,11.49 R27.2 22.6,11.4 | 22.6,11.4 | 22.6,11.4 22.54,11.34 R26.1 22.15,11.4 R25.1
N$30
  Bottom 0.508: Q5.E 17.29,9.91 15.96,11.24 R22.2
N$31
  Bottom 0.508: R23.2 11.01,11.21 10.4,10.6 10.52,10.48 Q6.E
N$32  (via drill 0.35 pad 0.8, 0.4)
  Top 0.508: v36.4,5.6 35.8,6.2 | 35.8,6.2 35.8,8.4 | 35.8,8.4 v36.4,9 | v24.2,5.4 24.2,8.6 25.4,9.8 v27.4,9.8 34.4,9.8 35.8,8.4 | 35.8,6.2 35.8,2.8 v36.4,2.2
  Bottom 0.508: D3.C 29.11,15.04 27.94,13.86 | 27.94,13.86 R28.1 | 27.94,13.86 27.94,11.65 R27.1 27.69,10.09 v27.4,9.8 | T4.B 37.47,5.6 v36.4,5.6 | v36.4,9 37.54,9 T5.B | C18.2 25.24,4.36 v24.2,5.4 | v36.4,2.2 36.57,2.03 T3.B
N$33
  Bottom 0.508: R29.1 34.95,10.87 T5.E
N$34
  Bottom 0.508: R31.1 37.74,3.94 T3.E
N$35
  Bottom 0.508: R32.2 48.36,2.62 D4.C 48.38,3.1 49.64,4.36 52.76,4.36 53.8,5.4 53.8,12.4 52.27,13.93 Q10.B
N$36  (via drill 0.35 pad 0.8)
  Top 0.508: v46.19,11.29 48.46,9.02 v51.07,9.02
  Bottom 0.508: Q8.C 46.17,11.31 v46.19,11.29 | v51.07,9.02 50.17,9.02 Q7.B 50.09,8.11 49.44,7.45 R33.1
N$37
  Bottom 0.508: Q10.C 49.14,17.96 R35.1
N$38
  Bottom 0.508: Q9.C 42.15,16.23 R37.2 42.2,18.64 R36.1
N$39
  Bottom 0.508: Q7.E Q8.B 45.55,6.23 R34.2
N$40  (via drill 0.35 pad 0.8)
  Top 0.508: v41.6,10.2 41.6,19 43.8,21.2 v48.2,21.2 | v47.6,33.2 47.6,32 50,29.6 v50,28.6
  Bottom 0.508: T3.C 41.6,4.63 | 41.6,4.63 41.6,6 | 41.6,6 41.6,6.4 | 41.6,6.4 41.6,8.2 | 41.6,8.2 41.4,8.4 | 41.4,8.4 39.88,9.92 T5.C | T4.C 41.52,6.47 41.6,6.4 | R34.1 41.69,6.09 41.6,6 | R32.1 41.8,4.63 41.6,4.63 | Q8.E 42.51,9.11 41.6,8.2 | v48.2,21.2 49.96,22.96 C19.2 49.93,24.46 R39.1 50,27.16 v50,28.6 | v41.6,10.2 41.6,8.6 41.4,8.4 | Q12.2 47.6,32.43 v47.6,33.2
N$41
  Bottom 0.508: R37.1 42.15,23.08 | 42.15,23.08 R38.2 | Q11.B 42.2,23.13 42.15,23.08
N$42
  Bottom 0.508: R39.2 48.03,24.46 C19.1 | R39.2 44.47,27.09 Q11.C | Q12.1 48.03,30.09 R39.2
N$43
  Bottom 0.508: Q7.C 48.19,12.25 Q10.E 48.15,13.97 Q9.E
N$44
  Top 0.3: U$2.5 66.41,20.61 65.2,19.4 62.8,19.4 62.05,18.65 Q13.2 C14.2
N$45
  Bottom 0.508: R42.1 49.95,35.15 Q12.3 53.48,27.79 R41.1
N$46  (via drill 0.35 pad 0.8)
  Top 0.508: v47.34,15.81 v51.99,15.81 v52,15.8
  Bottom 0.508: Q9.B 47.28,15.87 v47.34,15.81 | C17.1 55.91,16.72 R40.1 52.91,15.8 v52,15.8 52,20.52 R41.2
N$47
  Top 0.3: U$2.6 66.91,18.43 Q13.1 67,18.26 C15.2
N$48  (via drill 0.35 pad 0.8)
  Top 0.3: 55.71,27.34 R43.1 v57.39,27.39 v57.4,27.4 | v60.2,27.4 60.26,27.34 U$2.60
  Bottom 0.3: v57.4,27.4 v60.2,27.4
N$49
  Top 0.3: U$2.13 70.41,14.59 71.14,13.86 C28.2
  Top 0.508: R45.1 73.75,13.81 C28.2
N$50  (via drill 0.6)
  Top 0.508: v49.35,50.62 49.2,50.47 v49.2,46
  Bottom 0.508: Q15.1 50.66,43.5 R49.2 48.91,43.63 48.91,45.7 v49.2,46 | Q16.C v49.36,50.61 v49.35,50.62 | v49.2,46
N$51
  Top 0.508: Q14.B 61.31,4.65 61.31,3.4 | 61.31,3.4 R48.1 | FOTODIOD.2 61.31,3.4
N$52
  Bottom 0.406: D9.C
  Bottom 0.508: D2.A D9.C
NET
  Top 0.508: D7.A 63.22,10.64 R46.1 | R46.1 65.32,8.65 D8.C 65.35,10.18 R54.2 | Q14.E 62.33,6.73 63.22,7.62 R46.1
NRST  (via drill 0.35 pad 0.35)
  Top 0.3: U$2.7 67.41,24.99 65.8,26.6 v65.6,26.6 | v52.24,34.58 52.24,36.33 52.17,36.4 R44.1 52.2,39.05 52.2,47.2 54.42,49.42 PRG.5
  Top 0.508: 52.17,36.4 C16.1
  Bottom 0.3: v65.6,26.6 62.4,29.8 55.3,29.8 52.24,32.86 v52.24,34.58
NSS1  (via drill 0.35 pad 0.35)
  Top 0.3: U$2.20 79.23,26.84 v79.81,26.26
  Bottom 0.3: v79.81,26.26 79.81,17.79 81.4,16.2 87.61,16.2 DISPLAY-CON.3
RESETDSP  (via drill 0.35 pad 0.35)
  Top 0.3: U$2.43 66.91,26.89 v67.6,26.2 | v77.4,18.8 87.59,18.8 DISPLAY-CON.4
  Bottom 0.3: v67.6,26.2 75,18.8 v77.4,18.8
SCK1
  Top 0.3: U$2.21 82.08,27.34 83.04,26.38 DISPLAY-CON.7
SCL  (via drill 0.35 pad 0.35)
  Top 0.3: U$2.58 64.74,28.34 65.8,29.4 v65.8,32.2 | v76.6,49.2 76.54,49.26 R51.2
  Top 0.508: BME280.4 74.3,51.7 75.41,50.59 R51.2
  Bottom 0.3: v65.8,32.2 65.8,37.6 69,40.8 74.8,40.8 76.6,42.6 v76.6,49.2
SDA  (via drill 0.35 pad 0.35)
  Top 0.3: U$2.59 65.44,27.84 v66,28.4 | v68,38.2 71.4,38.2 73,39.8 v73,45.6 | v73,50.6 v72.99,50.59 R52.2
  Top 0.508: BME280.3 71.76,50.52 R52.2
  Bottom 0.3: v66,28.4 66.8,29.2 66.8,34.6 | 66.8,34.6 | 66.8,34.6 66.8,37 v68,38.2 | v73,45.6 v73,50.6
SDO
  Top 0.508: R53.1 66.68,50.93 BME280.1
SWCLK  (via drill 0.35 pad 0.35)
  Top 0.3: U$2.49 v62.41,35.59 v62.4,35.6
  Bottom 0.3: v62.4,35.6 62.4,44 59.52,46.88 PRG.4
SWDIO  (via drill 0.35 pad 0.35)
  Top 0.3: PRG.3 63.36,44.36 v63.4,44.4 | U$2.46 65.41,37.19 65.4,37.2 v65.4,38.8
  Bottom 0.3: v65.4,38.8 65.4,42.4 v63.4,44.4
VCC  (via drill 0.35 pad 0.8)
  Top 0.3: U$2.64 59.84,25.34 58.61,24.11 C10.2 | U$2.19 77.42,26.34 C12.2 | U$2.32 77.86,32.84 C13.1 | U$2.48 64.41,37.39 63.27,38.53 C11.2
  Top 0.508: 57.21,39 59,39 60.6,40.6 C11.2 63.27,41.87 64.4,43 v71,43 | 57.21,39 PRG.1 56.97,30.83 58.6,29.2 58.6,22.81 58.6,22.8 | R44.2 57.19,39.02 57.21,39 | Q14.C 58.59,6.13 v58.59,8 v58.59,10.2 D7.C 58.59,20.55 58.6,22.8 | 73.75,9.01 R45.2 | R45.2 85.72,9.23 DISPLAY-CON.1 | FOTODIOD.1 67.73,4.87 v66.2,6.4 | v72.4,9.2 73.72,9.2 R45.2 | 58.6,22.8 C10.2 | v74.4,43 78.41,38.99 C13.1 v78.41,31.01 v78.4,31 | v78.4,23.2 79.15,23.95 C12.2
  Bottom 0.508: C8.+ 44.15,48.6 | 44.15,48.6 44.15,42.9 C7.+ 44.2,38.98 C6.1 44.47,37.26 D6.C 46.92,35.32 R42.2 47.03,37.43 48.6,39 54.4,39 56.73,39 PRG.1 | v66.2,6.4 60.19,6.4 v58.59,8 | v58.59,10.2 59.59,9.2 v72.4,9.2 | v71,43 v74.4,43 | v78.4,31 v78.4,23.2 | Q16.E 48.41,48.19 47.4,49.2 | R47.2 47.8,52.3 47.8,49.6 47.7,49.5 47.4,49.2 | 44.15,48.6 46.8,48.6 47.4,49.2
VDD  (via drill 0.35 pad 0.8)
  Top 0.508: R56.1 | R56.1 69.66,48.94 71.21,47.39 R52.1 75.38,47.39 R51.1 75.45,47.4 77,47.4 77.8,48.2 C21.1 79.68,48.23 C20.1 79.38,50.79 BME280.6 | v69.4,47.6 R56.1
  Bottom 0.508: Q15.3 53.47,50.67 55,52.2 62.4,52.2 64.2,50.4 64.2,46.6 65.8,45 68.2,45 69.4,46.2 v69.4,47.6
WRITEDSP  (via drill 0.35 pad 0.35)
  Top 0.3: U$2.42 67.41,28.19 v69.2,26.4 | v78,21.6 87.33,21.6 DISPLAY-CON.5
  Bottom 0.3: v69.2,26.4 74,21.6 v78,21.6

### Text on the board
tNames: LN-Electronic | WS-01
